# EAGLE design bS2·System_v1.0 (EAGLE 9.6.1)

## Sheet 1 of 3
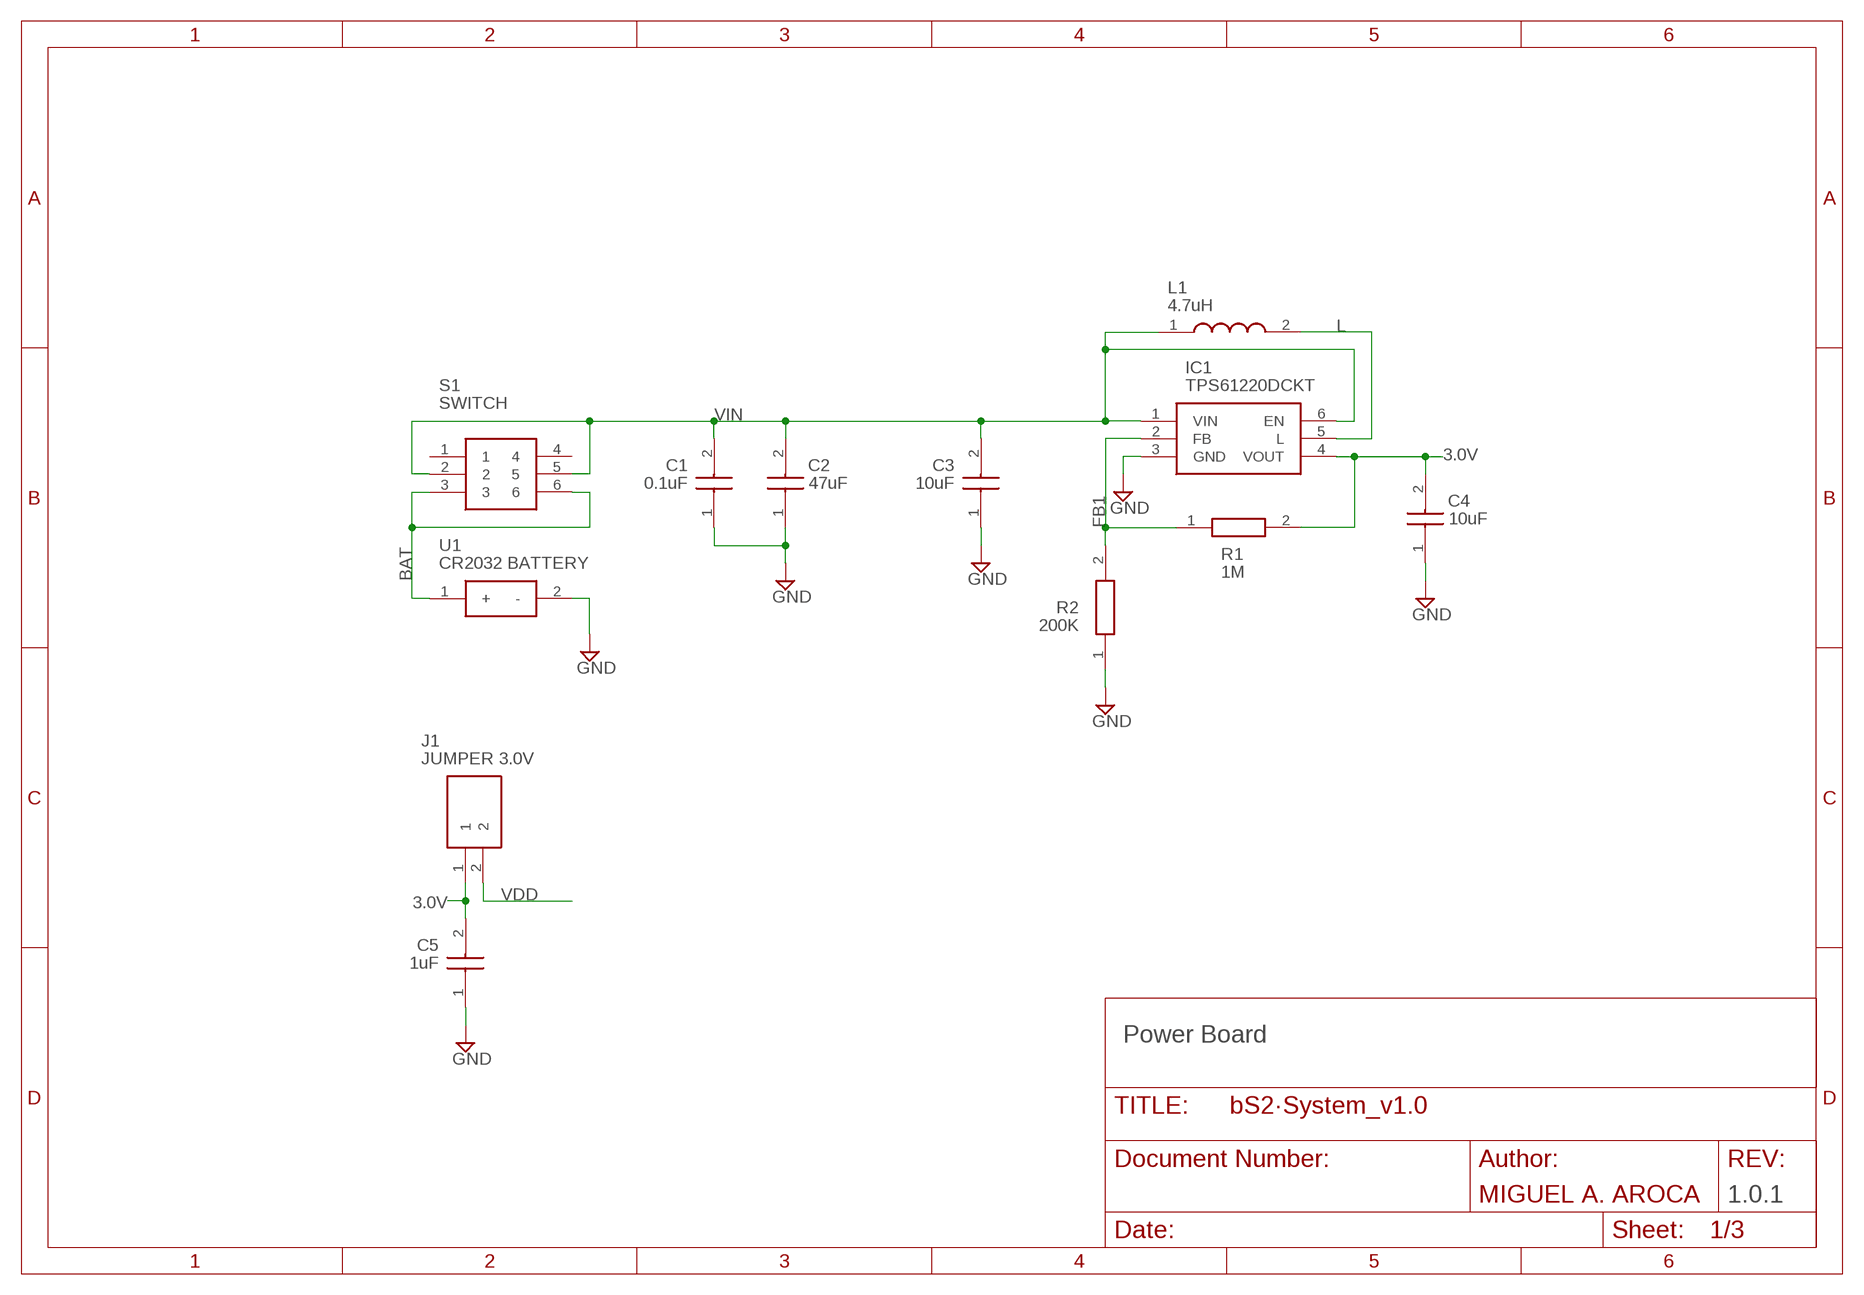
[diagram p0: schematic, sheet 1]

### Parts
C1  0.1uF  C0402C104K4RAC7411  [CAPC1005X55N]
C2  47uF  C1210C476K8RACTU  [CAPC3225X280N]
C3  10uF  GRM188R60J106ME84D  [CAPC1608X90N]
C4  10uF  GRM188R60J106ME84D  [CAPC1608X90N]
C5  1uF  0603ZC105KAT2A  [CAPC1608X90N]
IC1  TPS61220DCKT  [SOT65P210X110-6N]
J1  JUMPER 3.0V  22-28-4027  [HDRV2W66P0X254_1X2_508X249X106]
L1  4.7uH  EPL3015-472MLB  [INDC3030X155N]
R1  1M  CR0402-FX-1004GLF  [RESC1005X40N]
R2  200K  CR0402-JW-204GLF  [RESC1005X40N]
S1  SWITCH  JS202011SCQN  [JS202011SCQN]
U1  CR2032 BATTERY  SMTU2032-LF  [SMTU2032LF]

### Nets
3.0V: C4.2 C5.2 IC1.4(VOUT) J1.1 R1.2
BAT: S1.3 S1.6 U1.1(+)
FB1: IC1.2(FB) R1.1 R2.2
GND: C1.1 C2.1 C3.1 C4.1 C5.1 IC1.3(GND) R2.1 U1.2(-) ; also sheet 2,3
L: IC1.5(L) L1.2
VDD: J1.2 ; also sheet 2,3
VIN: C1.2 C2.2 C3.2 IC1.1(VIN) IC1.6(EN) L1.1 S1.2 S1.5
Unconnected: S1.1 S1.4

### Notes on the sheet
- Power Board
- 1.0.1

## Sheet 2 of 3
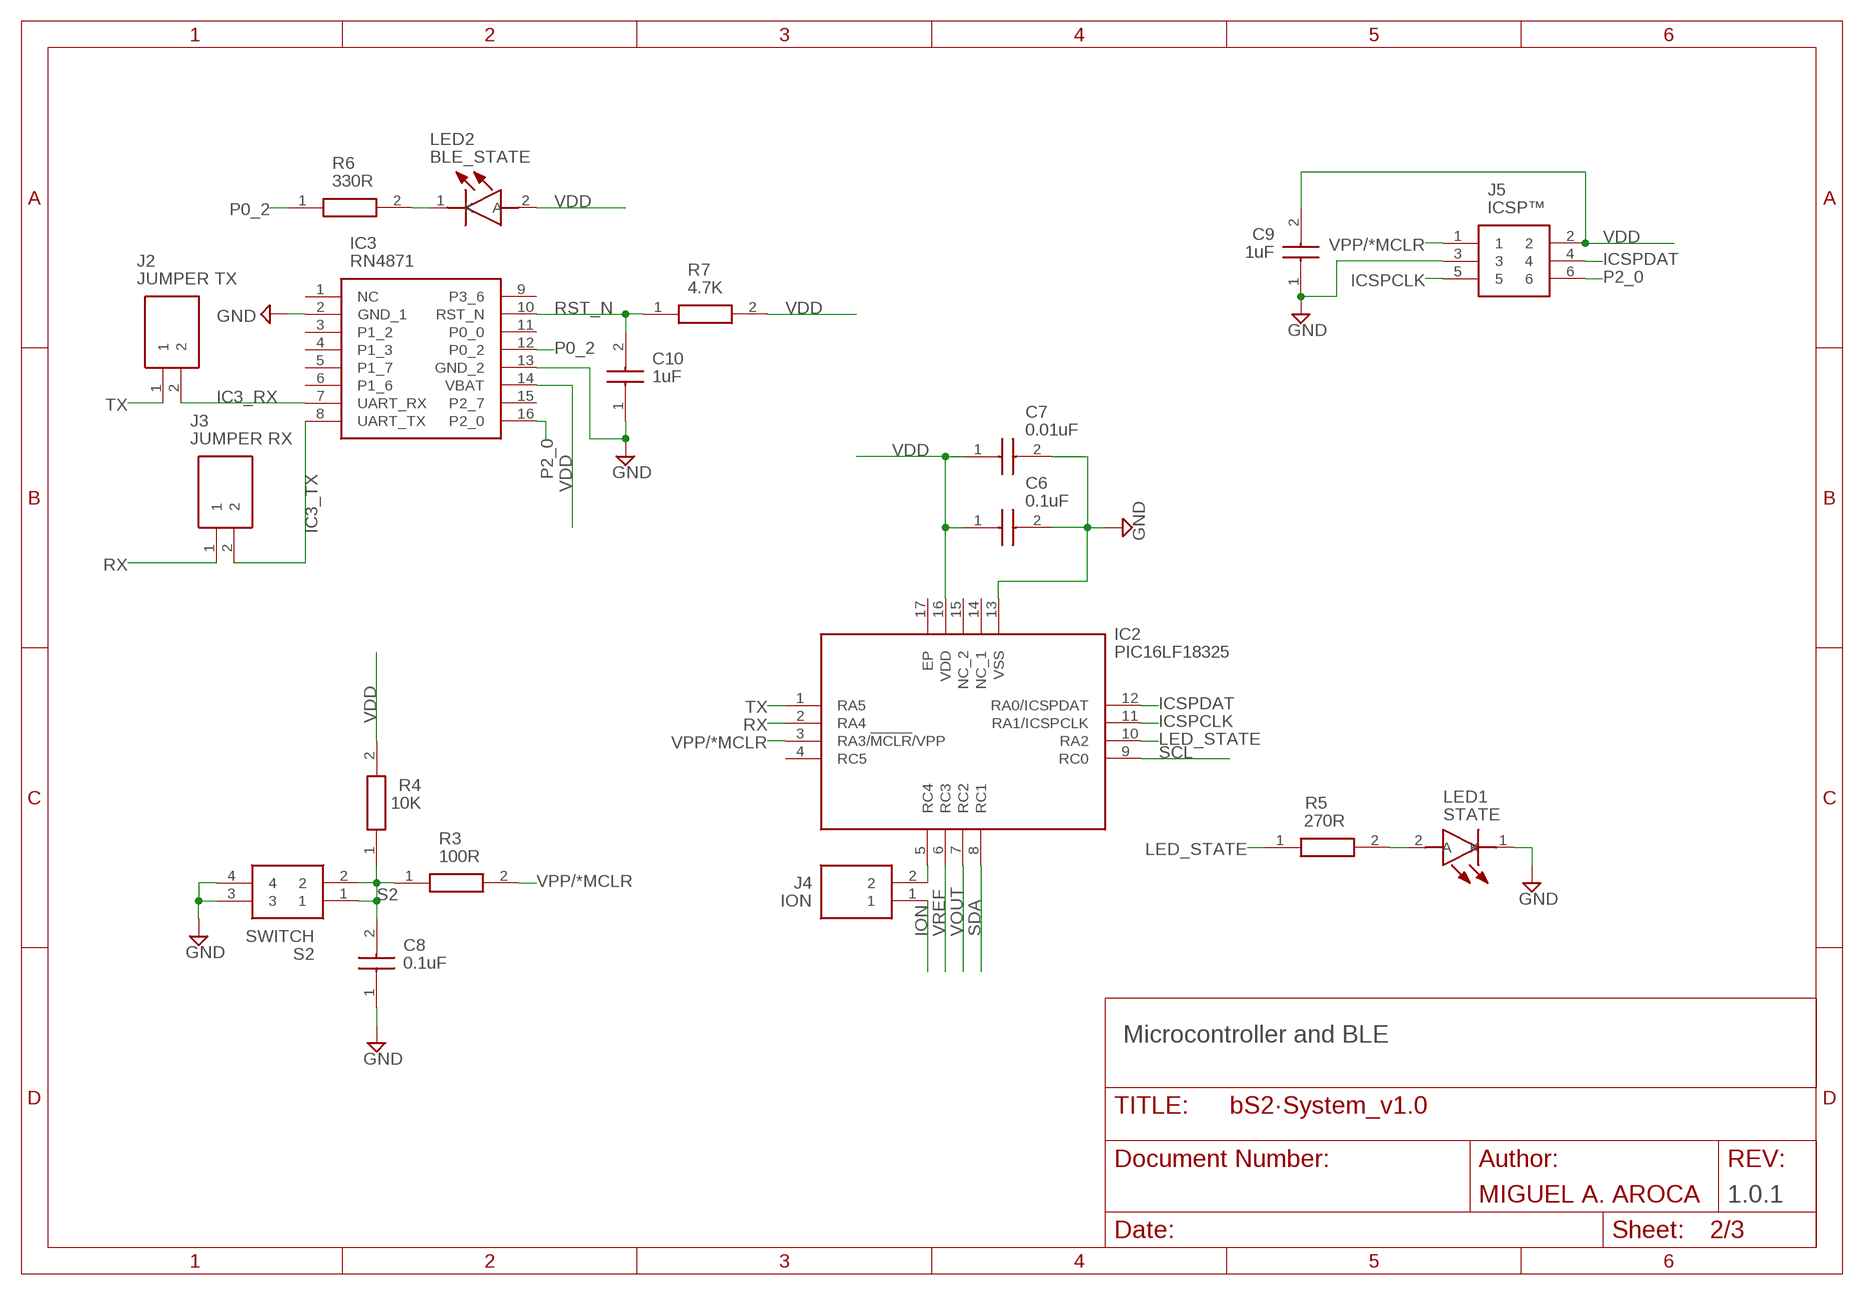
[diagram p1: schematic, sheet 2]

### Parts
C6  0.1uF  C0402C104K4RAC7411  [CAPC1005X55N]
C7  0.01uF  0402ZC103JAT2A  [CAPC1005X56N]
C8  0.1uF  C0402C104K4RAC7411  [CAPC1005X55N]
C9  1uF  0603ZC105KAT2A  [CAPC1608X90N]
C10  1uF  0603ZC105KAT2A  [CAPC1608X90N]
IC2  PIC16LF18325  PIC16LF18325-I_JQ  [QFN65P400X400X55-17N]
IC3  RN4871  RN4871-I_RM130  [RN4871]
J2  JUMPER TX  22-28-4027  [HDRV2W66P0X254_1X2_508X249X106]
J3  JUMPER RX  22-28-4027  [HDRV2W66P0X254_1X2_508X249X106]
J4  ION  22-28-4027  [HDRV2W66P0X254_1X2_508X249X106]
J5  ICSP™  87898-0666  [878980666]
LED1  STATE  SMLP12BC7TT86  [LEDC1006X25N]
LED2  BLE_STATE  SMLP12BC7TT86  [LEDC1006X25N]
R3  100R  CR0402-JW-101GLF  [RESC1005X40N]
R4  10K  CRCW040210K0FKED  [RESC1005X40N]
R5  270R  CR0402-JW-271GLF  [RESC1005X40N]
R6  330R  CR0402-JW-331GLF  [RESC1005X40N]
R7  4.7K  CR0402-JW-472GLF  [RESC1005X40N]
S2  SWITCH  SKRPANE010  [SKRPADE010]

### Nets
GND: C6.2 C7.2 C8.1 C9.1 C10.1 IC2.13(VSS) IC3.2(GND_1) IC3.13(GND_2) J5.3 LED1.1(K) S2.3 S2.4 ; also sheet 1,3
IC3_RX: IC3.7(UART_RX) J2.2
IC3_TX: IC3.8(UART_TX) J3.2
ICSPCLK: IC2.11(RA1/ICSPCLK) J5.5
ICSPDAT: IC2.12(RA0/ICSPDAT) J5.4
ION: J4.1 ; also sheet 3
LED1: LED1.2(A) R5.2
LED2_K: LED2.1(K) R6.2
LED_STATE: IC2.10(RA2) R5.1
P0_2: IC3.12(P0_2) R6.1
P2_0: IC3.16(P2_0) J5.6
RC4: IC2.5(RC4) J4.2
RST_N: C10.2 IC3.10(RST_N) R7.1
RX: IC2.2(RA4) J3.1
S2: C8.2 R3.1 R4.1 S2.1 S2.2
SCL: IC2.9(RC0) ; also sheet 3
SDA: IC2.8(RC1) ; also sheet 3
TX: IC2.1(RA5) J2.1
VDD: C6.1 C7.1 C9.2 IC2.16(VDD) IC3.14(VBAT) J5.2 LED2.2(A) R4.2 R7.2 ; also sheet 1,3
VOUT: IC2.7(RC2) ; also sheet 3
VPP/*MCLR: IC2.3(RA3/!MCLR!/VPP) J5.1 R3.2
VREF: IC2.6(RC3) ; also sheet 3
Unconnected: IC2.4(RC5) IC2.14(NC_1) IC2.15(NC_2) IC2.17(EP) IC3.1(NC) IC3.3(P1_2) IC3.4(P1_3) IC3.5(P1_7) IC3.6(P1_6) IC3.9(P3_6) IC3.11(P0_0) IC3.15(P2_7)

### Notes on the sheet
- Microcontroller and BLE
- 1.0.1

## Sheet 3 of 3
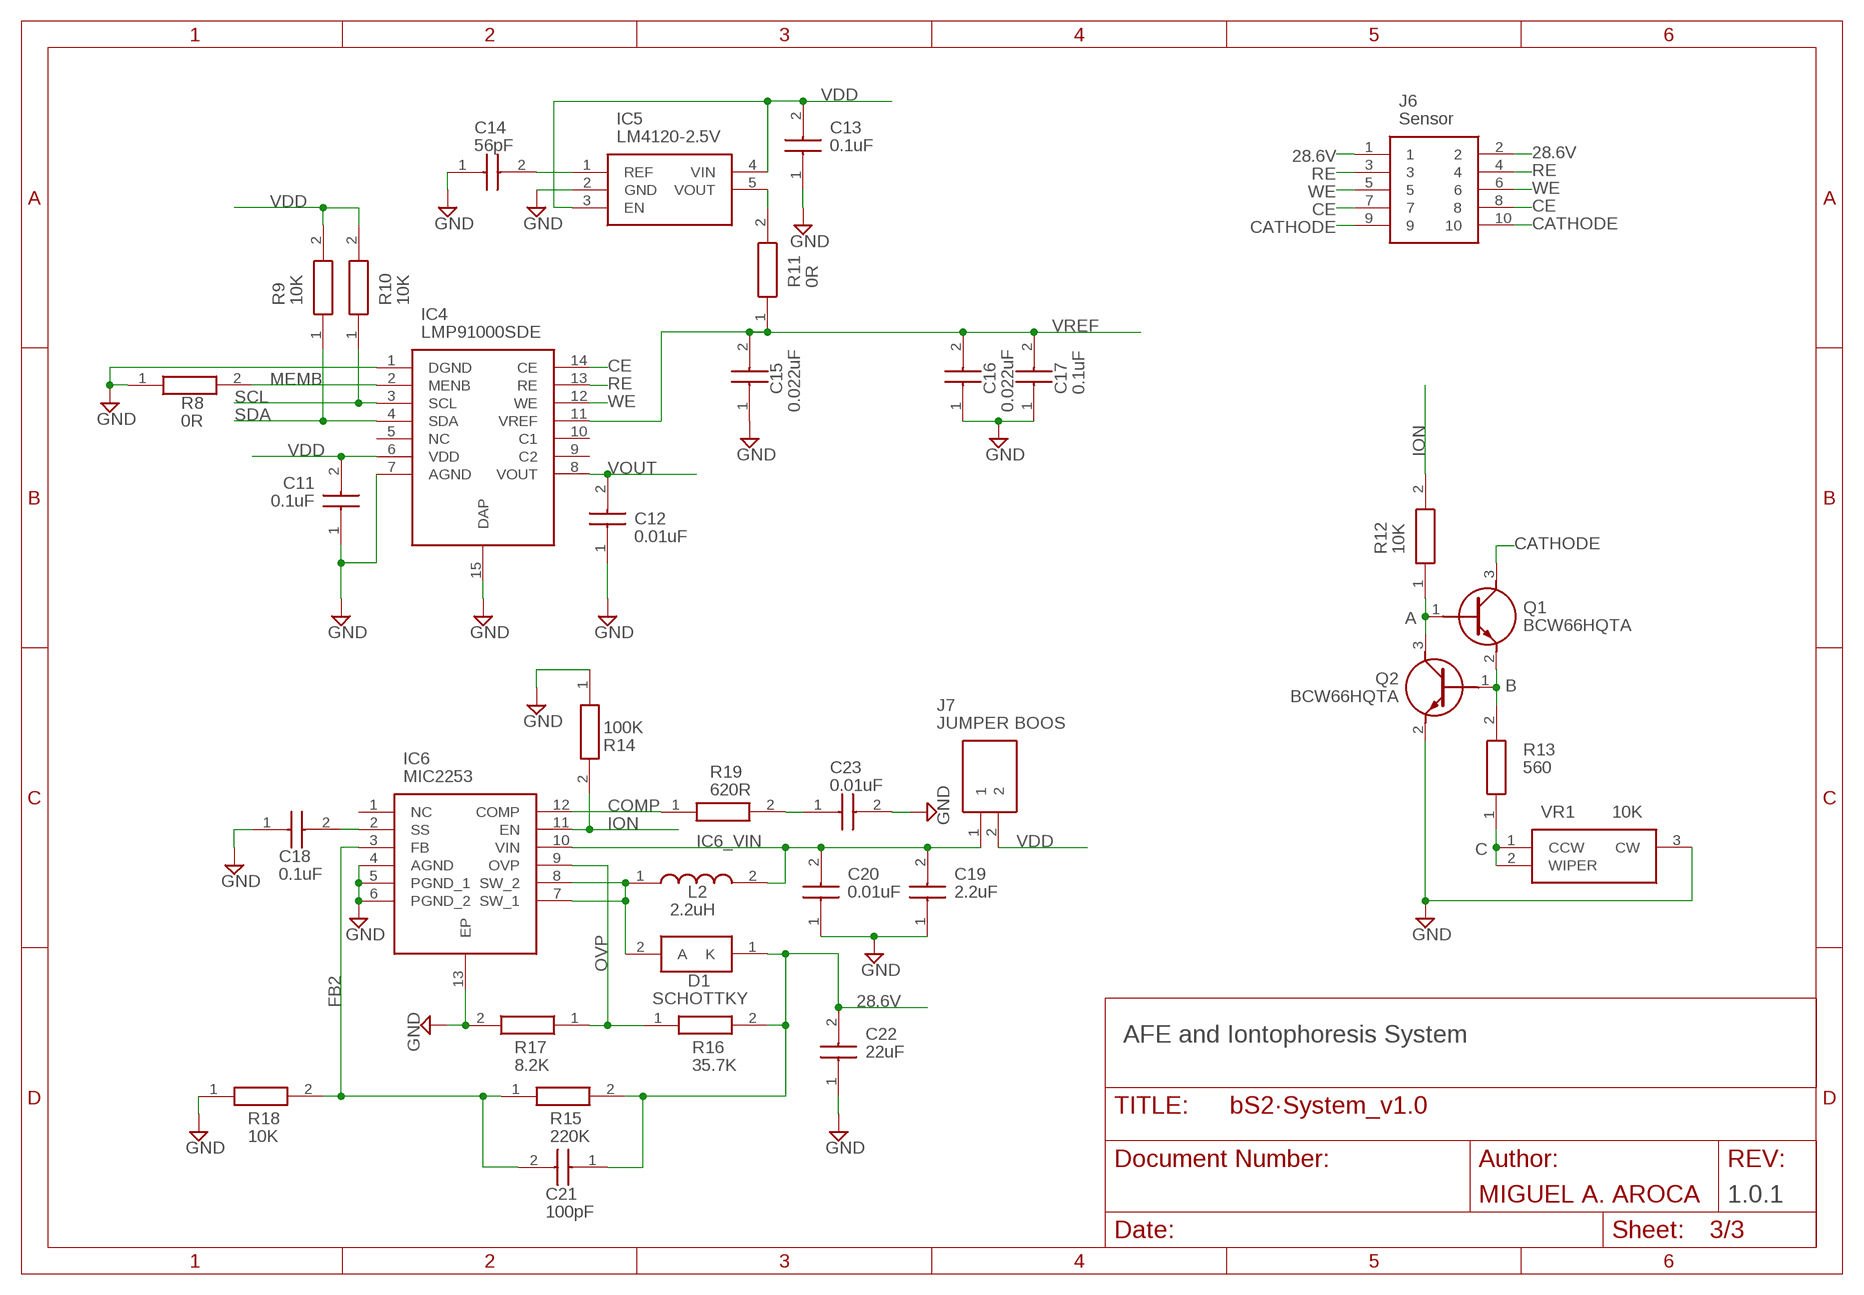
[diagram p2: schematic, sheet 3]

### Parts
C11  0.1uF  C0402C104K4RAC7411  [CAPC1005X55N]
C12  0.01uF  0402ZC103JAT2A  [CAPC1005X56N]
C13  0.1uF  C0402C104K4RAC7411  [CAPC1005X55N]
C14  56pF  VJ0402D560JXAAJ  [CAPC1005X61N]
C15  0.022uF  C0402C223K4RACTU  [CAPC1005X55N]
C16  0.022uF  C0402C223K4RACTU  [CAPC1005X55N]
C17  0.1uF  C0402C104K4RAC7411  [CAPC1005X55N]
C18  0.1uF  CGA2B3X7R1H104K050BE  [CAPC1005X55N]
C19  2.2uF  GRM188R61H225KE11D  [CAPC1608X90N]
C20  0.01uF  C1005X7R1H103K050BE  [CAPC1005X55N]
C21  100pF  C0402C101F5GAC  [CAPC1005X55N]
C22  22uF  C3216X5R1V226M160AC  [CAPC3216X180N]
C23  0.01uF  C1005X7R1H103K050BE  [CAPC1005X55N]
D1  SCHOTTKY  SSA24-E3_61T  [DIONM5127X229N]
IC4  LMP91000SDE  LMP91000SDE_NOPB  [SON50P400X400X80-15N]
IC5  LM4120-2.5V  LM4120AIM5-2.5_NOPB  [SOT95P280X145-5N]
IC6  MIC2253  MIC2253-06YML-TR  [SON50P300X300X90-13N]
J6  Sensor  39-53-2104  [39532104]
J7  JUMPER BOOS  22-28-4027  [HDRV2W66P0X254_1X2_508X249X106]
L2  2.2uH  XAL4020-222MEC  [XAL40XX]
Q1  BCW66HQTA  [FMMT619TA]
Q2  BCW66HQTA  [FMMT619TA]
R8  0R  ERJ-2GE0R00X  [RESC1005X40N]
R9  10K  CRCW040210K0FKED  [RESC1005X40N]
R10  10K  CRCW040210K0FKED  [RESC1005X40N]
R11  0R  ERJ-2GE0R00X  [RESC1005X40N]
R12  10K  CRCW040210K0FKED  [RESC1005X40N]
R13  560  CR0402-JW-561GLF  [RESC1005X40N]
R14  100K  ERJ-3EKF1003V  [RESC1608X55N]
R15  220K  ERJ-3EKF2203V  [RESC1608X55N]
R16  35.7K  ERJ-3EKF3572V  [RESC1608X55N]
R17  8.2K  ERJ-3EKF8201V  [RESC1608X55N]
R18  10K  ERJ-3EKF1002V  [RESC1608X55N]
R19  620R  ERJ-3EKF6200V  [RESC1608X55N]
VR1  10K  3224W-1-103E  [3224W1205E]

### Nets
28.6V: C21.1 C22.2 D1.1(K) J6.1 J6.2 R15.2 R16.2
A: Q1.1(B) Q2.3(C) R12.1
B: Q1.2(E) Q2.1(B) R13.2
C: R13.1 VR1.1(CCW) VR1.2(WIPER)
CATHODE: J6.9 J6.10 Q1.3(C)
CE: IC4.14(CE) J6.7 J6.8
COMP: IC6.12(COMP) R19.1
COMP*: C23.1 R19.2
FB2: C21.2 IC6.3(FB) R15.1 R18.2
GND: C11.1 C12.1 C13.1 C14.1 C15.1 C16.1 C17.1 C18.1 C19.1 C20.1 C22.1 C23.2 IC4.1(DGND) IC4.7(AGND) IC4.15(DAP) IC5.2(GND) IC6.4(AGND) IC6.5(PGND_1) IC6.6(PGND_2) IC6.13(EP) Q2.2(E) R8.1(R1) R14.1 R17.2 R18.1 VR1.3(CW) ; also sheet 1,2
IC5_OUT: IC5.5(VOUT) R11.2(R2)
IC5_REF: C14.2 IC5.1(REF)
IC6_VIN: C19.2 C20.2 IC6.10(VIN) J7.1 L2.2
ION: IC6.11(EN) R12.2 R14.2 ; also sheet 2
MEMB: IC4.2(MENB) R8.2(R2)
OVP: IC6.9(OVP) R16.1 R17.1
RE: IC4.13(RE) J6.3 J6.4
SCL: IC4.3(SCL) R10.1 ; also sheet 2
SDA: IC4.4(SDA) R9.1 ; also sheet 2
SS: C18.2 IC6.2(SS)
SW: D1.2(A) IC6.7(SW_1) IC6.8(SW_2) L2.1
VDD: C11.2 C13.2 IC4.6(VDD) IC5.3(EN) IC5.4(VIN) J7.2 R9.2 R10.2 ; also sheet 1,2
VOUT: C12.2 IC4.8(VOUT) ; also sheet 2
VREF: C15.2 C16.2 C17.2 IC4.11(VREF) R11.1(R1) ; also sheet 2
WE: IC4.12(WE) J6.5 J6.6
Unconnected: IC4.5(NC) IC4.9(C2) IC4.10(C1) IC6.1(NC)

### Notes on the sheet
- AFE and Iontophoresis System
- 1.0.1

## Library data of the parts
C1 C6 C8 C11 C13 C17 = SamacSys_Parts:C0402C104K4RAC7411: Multilayer Ceramic Capacitors MLCC - SMD/SMT 16V 0.1uF X7R 0402 10%; DESCRIPTION: Multilayer Ceramic Capacitors MLCC - SMD/SMT 16V 0.1uF X7R 0402 10%; HEIGHT: 0.55mm; MANUFACTURER_NAME: Kemet; MANUFACTURER_PART_NUMBER: C0402C104K4RAC7411; MOUSER_PART_NUMBER: 80-C0402C104K4R7411; MOUSER_PRICE-STOCK: https://www.mouser.com/Search/Refine.aspx?Keyword=80-C0402C104K4R7411; RS_PART_NUMBER: 1806459; RS_PRICE-STOCK: http://uk.rs-online.com/web/p/products/1806459
C2 = SamacSys_Parts:C1210C476K8RACTU: Multilayer Ceramic Capacitors MLCC - SMD/SMT 10volts 47uF 10% X7R; DESCRIPTION: Multilayer Ceramic Capacitors MLCC - SMD/SMT 10volts 47uF 10% X7R; HEIGHT: 2.8mm; MANUFACTURER_NAME: Kemet; MANUFACTURER_PART_NUMBER: C1210C476K8RACTU; MOUSER_PART_NUMBER: 80-C1210C476K8R; MOUSER_PRICE-STOCK: https://www.mouser.com/Search/Refine.aspx?Keyword=80-C1210C476K8R; RS_PART_NUMBER: 1611519P; RS_PRICE-STOCK: http://uk.rs-online.com/web/p/products/1611519P
C3 C4 = SamacSys_Parts:GRM188R60J106ME84D: Multilayer Ceramic Capacitors MLCC - SMD/SMT 0603 10uF 6.3volts X5R 20%; DESCRIPTION: Multilayer Ceramic Capacitors MLCC - SMD/SMT 0603 10uF 6.3volts X5R 20%; HEIGHT: 0.9mm; MANUFACTURER_NAME: Murata Electronics; MANUFACTURER_PART_NUMBER: GRM188R60J106ME84D; MOUSER_PART_NUMBER: 81-GRM188R60J106ME4D; MOUSER_PRICE-STOCK: https://www.mouser.com/Search/Refine.aspx?Keyword=81-GRM188R60J106ME4D; RS_PART_NUMBER: 8847242P; RS_PRICE-STOCK: http://uk.rs-online.com/web/p/products/8847242P
C5 C9 C10 = SamacSys_Parts:0603ZC105KAT2A: AVX - 0603ZC105KAT2A - CAP, MLCC, X7R, 1UF, 10V, 0603; DESCRIPTION: AVX - 0603ZC105KAT2A - CAP, MLCC, X7R, 1UF, 10V, 0603; HEIGHT: 0.9mm; MANUFACTURER_NAME: AVX; MANUFACTURER_PART_NUMBER: 0603ZC105KAT2A; MOUSER_PART_NUMBER: 581-0603ZC105KAT2A; MOUSER_PRICE-STOCK: https://www.mouser.com/Search/Refine.aspx?Keyword=581-0603ZC105KAT2A; RS_PART_NUMBER: 1358373; RS_PRICE-STOCK: http://uk.rs-online.com/web/p/products/1358373
C7 C12 = SamacSys_Parts:0402ZC103JAT2A: Multilayer Ceramic Capacitors MLCC - SMD/SMT 10V .01uF X7R 0402 5%; DESCRIPTION: Multilayer Ceramic Capacitors MLCC - SMD/SMT 10V .01uF X7R 0402 5%; HEIGHT: 0.56mm; MANUFACTURER_NAME: AVX; MANUFACTURER_PART_NUMBER: 0402ZC103JAT2A; MOUSER_PART_NUMBER: 581-0402ZC103JAT2A; MOUSER_PRICE-STOCK: https://www.mouser.com/Search/Refine.aspx?Keyword=581-0402ZC103JAT2A
C14 = SamacSys_Parts:VJ0402D560JXAAJ: Multilayer Ceramic Capacitors MLCC - SMD/SMT 0402 56pF 50V C0G 5% HI FREQ; DESCRIPTION: Multilayer Ceramic Capacitors MLCC - SMD/SMT 0402 56pF 50V C0G 5% HI FREQ; HEIGHT: 0.61mm; MANUFACTURER_NAME: VISHAY VITRAMON; MANUFACTURER_PART_NUMBER: VJ0402D560JXAAJ
C15 C16 = SamacSys_Parts:C0402C223K4RACTU: Kemet 1005 C0402C 22nF Ceramic Multilayer Capacitor, 16 V dc, +125C, X7R Dielectric, +/-10%; DESCRIPTION: Kemet 1005 C0402C 22nF Ceramic Multilayer Capacitor, 16 V dc, +125C, X7R Dielectric, +/-10%; HEIGHT: 0.55mm; MANUFACTURER_NAME: Kemet; MANUFACTURER_PART_NUMBER: C0402C223K4RACTU; MOUSER_PART_NUMBER: 80-C0402C223K4R; MOUSER_PRICE-STOCK: https://www.mouser.com/Search/Refine.aspx?Keyword=80-C0402C223K4R; RS_PART_NUMBER: 0147724; RS_PRICE-STOCK: http://uk.rs-online.com/web/p/products/0147724
C18 = SamacSys_Parts:CGA2B3X7R1H104K050BE: Multilayer Ceramic Capacitors MLCC - SMD/SMT 0402 0.1uF 50volts X7R 10% Soft Term; DESCRIPTION: Multilayer Ceramic Capacitors MLCC - SMD/SMT 0402 0.1uF 50volts X7R 10% Soft Term; HEIGHT: 0.55mm; MANUFACTURER_NAME: TDK; MANUFACTURER_PART_NUMBER: CGA2B3X7R1H104K050BE; MOUSER_PART_NUMBER: 810-CGA2B3X7R1H104KB; MOUSER_PRICE-STOCK: https://www.mouser.com/Search/Refine.aspx?Keyword=810-CGA2B3X7R1H104KB
C19 = SamacSys_Parts:GRM188R61H225KE11D: Murata 1608 GRM 2200nF Ceramic Multilayer Capacitor, 50 V dc, +85C, X5R Dielectric, +/-10%; DESCRIPTION: Murata 1608 GRM 2200nF Ceramic Multilayer Capacitor, 50 V dc, +85C, X5R Dielectric, +/-10%; HEIGHT: 0.9mm; MANUFACTURER_NAME: Murata Electronics; MANUFACTURER_PART_NUMBER: GRM188R61H225KE11D; MOUSER_PART_NUMBER: 81-GRM188R61H225KE1D; MOUSER_PRICE-STOCK: https://www.mouser.com/Search/Refine.aspx?Keyword=81-GRM188R61H225KE1D; RS_PART_NUMBER: 8847289P; RS_PRICE-STOCK: http://uk.rs-online.com/web/p/products/8847289P
C20 C23 = SamacSys_Parts:C1005X7R1H103K050BE: Multilayer Ceramic Capacitors MLCC - SMD/SMT 0402 0.01uF 50volts X7R 10% Soft Term; DESCRIPTION: Multilayer Ceramic Capacitors MLCC - SMD/SMT 0402 0.01uF 50volts X7R 10% Soft Term; HEIGHT: 0.55mm; MANUFACTURER_NAME: TDK; MANUFACTURER_PART_NUMBER: C1005X7R1H103K050BE; MOUSER_PART_NUMBER: 810-C1005X7R1H103KBE; MOUSER_PRICE-STOCK: https://www.mouser.com/Search/Refine.aspx?Keyword=810-C1005X7R1H103KBE
C21 = SamacSys_Parts:C0402C101F5GAC: Multilayer Ceramic Capacitors MLCC - SMD/SMT 50volts 100pF 1% C0G; DESCRIPTION: Multilayer Ceramic Capacitors MLCC - SMD/SMT 50volts 100pF 1% C0G; HEIGHT: 0.55mm; MANUFACTURER_NAME: Kemet; MANUFACTURER_PART_NUMBER: C0402C101F5GAC; MOUSER_PART_NUMBER: 80-C0402C101F5GAC; MOUSER_PRICE-STOCK: https://www.mouser.com/Search/Refine.aspx?Keyword=80-C0402C101F5GAC
C22 = SamacSys_Parts:C3216X5R1V226M160AC: Multilayer Ceramic Capacitors MLCC - SMD/SMT 1206 22uF 35volts X5R 20%; DESCRIPTION: Multilayer Ceramic Capacitors MLCC - SMD/SMT 1206 22uF 35volts X5R 20%; HEIGHT: 1.8mm; MANUFACTURER_NAME: TDK; MANUFACTURER_PART_NUMBER: C3216X5R1V226M160AC; MOUSER_PART_NUMBER: 810-C3216X5R1V226M; MOUSER_PRICE-STOCK: https://www.mouser.com/Search/Refine.aspx?Keyword=810-C3216X5R1V226M; RS_PART_NUMBER: 7883063P; RS_PRICE-STOCK: http://uk.rs-online.com/web/p/products/7883063P
D1 = SamacSys_Parts:SSA24-E3_61T: Vishay 40V 2A, Diode, 2-Pin DO-214AC SSA24-E3/61T; ALLIED_NUMBER: R1082641; ALLIED_PRICE-STOCK: https://www.alliedelec.com/vishaydale-ssa24-e3-61t/R1082641/; DESCRIPTION: Vishay 40V 2A, Diode, 2-Pin DO-214AC SSA24-E3/61T; HEIGHT: 2.29mm; MANUFACTURER_NAME: Vishay; MANUFACTURER_PART_NUMBER: SSA24-E3/61T; MOUSER_PART_NUMBER: 625-SSA24-E3; MOUSER_PRICE-STOCK: https://www.mouser.com/Search/Refine.aspx?Keyword=625-SSA24-E3; RS_PART_NUMBER: 7103819P; RS_PRICE-STOCK: http://uk.rs-online.com/web/p/products/7103819P
IC1 = SamacSys_Parts:TPS61220DCKT: TPS61220DCKT, Boost Converter, Step Up 0.5A Adjustable, 1.8 5.5 V, 2000 kHz, 6-Pin SC-70 Source: Datasheet; DESCRIPTION: TPS61220DCKT, Boost Converter, Step Up 0.5A Adjustable, 1.8 5.5 V, 2000 kHz, 6-Pin SC-70; HEIGHT: 1.1mm; MANUFACTURER_NAME: Texas Instruments; MANUFACTURER_PART_NUMBER: TPS61220DCKT; MOUSER_PART_NUMBER: 595-TPS61220DCKT; MOUSER_PRICE-STOCK: https://www.mouser.com/Search/Refine.aspx?Keyword=595-TPS61220DCKT; RS_PART_NUMBER: 7094642P; RS_PRICE-STOCK: http://uk.rs-online.com/web/p/products/7094642P
IC2 = SamacSys_Parts:PIC16LF18325-I_JQ: Microchip Technology PIC16LF18325-I/JQ, 8bit 8 bit CPU Microcontroller, 32MHz, 14 kB Flash, 16-Pin UQFN Source: Datasheet; DESCRIPTION: Microchip Technology PIC16LF18325-I/JQ, 8bit 8 bit CPU Microcontroller, 32MHz, 14 kB Flash, 16-Pin UQFN; HEIGHT: 0.55mm; MANUFACTURER_NAME: Microchip; MANUFACTURER_PART_NUMBER: PIC16LF18325-I/JQ; MOUSER_PART_NUMBER: 579-PIC16LF18325I/JQ; MOUSER_PRICE-STOCK: https://www.mouser.com/Search/Refine.aspx?Keyword=579-PIC16LF18325I%2FJQ; RS_PART_NUMBER: 1772711P; RS_PRICE-STOCK: http://uk.rs-online.com/web/p/products/1772711P
IC3 = SamacSys_Parts:RN4871-I_RM130: Bluetooth BLE Module, Shielded, Antenna, Source: Datasheet; DESCRIPTION: Bluetooth BLE Module, Shielded, Antenna,; HEIGHT: mm; MANUFACTURER_NAME: Microchip; MANUFACTURER_PART_NUMBER: RN4871-I/RM130; MOUSER_PART_NUMBER: 579-RN4871IRM130; MOUSER_PRICE-STOCK: https://www.mouser.com/Search/Refine.aspx?Keyword=579-RN4871IRM130; RS_PART_NUMBER: 1765558P; RS_PRICE-STOCK: http://uk.rs-online.com/web/p/products/1765558P
IC4 = SamacSys_Parts:LMP91000SDE_NOPB: Texas Instruments,LMP91000SDE/NOPB,AFE LMP91000SDE/NOPB, Analogue Front End IC, 1-channel Serial-I2C, 14-Pin WSON Source: Datasheet; DESCRIPTION: Texas Instruments,LMP91000SDE/NOPB,AFE LMP91000SDE/NOPB, Analogue Front End IC, 1-channel Serial-I2C, 14-Pin WSON; HEIGHT: 0.8mm; MANUFACTURER_NAME: Texas Instruments; MANUFACTURER_PART_NUMBER: LMP91000SDE/NOPB; MOUSER_PART_NUMBER: 926-LMP91000SDE/NOPB; MOUSER_PRICE-STOCK: https://www.mouser.com/Search/Refine.aspx?Keyword=926-LMP91000SDE%2FNOPB; RS_PART_NUMBER: 7988774P; RS_PRICE-STOCK: http://uk.rs-online.com/web/p/products/7988774P
IC5 = SamacSys_Parts:LM4120AIM5-2.5_NOPB: 0.2% 50ppm/C Drift Precision Series Voltage Reference with Shutdown Enable Source: Datasheet; DESCRIPTION: 0.2% 50ppm/C Drift Precision Series Voltage Reference with Shutdown Enable; HEIGHT: 1.45mm; MANUFACTURER_NAME: Texas Instruments; MANUFACTURER_PART_NUMBER: LM4120AIM5-2.5/NOPB; MOUSER_PART_NUMBER: 926-LM4120AIM525NOPB; MOUSER_PRICE-STOCK: https://www.mouser.com/Search/Refine.aspx?Keyword=926-LM4120AIM525NOPB; RS_PART_NUMBER: 6394496; RS_PRICE-STOCK: https://uk.rs-online.com/web/p/products/6394496
IC6 = SamacSys_Parts:MIC2253-06YML-TR: 3.5A 1MHz Efficiency Boost Regulator Source: Datasheet; DESCRIPTION: 3.5A 1MHz Efficiency Boost Regulator; HEIGHT: 0.9mm; MANUFACTURER_NAME: Microchip; MANUFACTURER_PART_NUMBER: MIC2253-06YML-TR; MOUSER_PART_NUMBER: 998-MIC2253-06YMLTR; RS_PART_NUMBER: 9101638P; RS_PRICE-STOCK: http://uk.rs-online.com/web/p/products/9101638P
J1-J4 J7 = SamacSys_Parts:22-28-4027: Headers & Wire Housings VERT B/A HDR 2P; ALLIED_NUMBER: 71457608; ALLIED_PRICE-STOCK: https://www.alliedelec.com/molexincorporated-22-28-4027/71457608/; DESCRIPTION: Headers & Wire Housings VERT B/A HDR 2P; HEIGHT: 10.67mm; MANUFACTURER_NAME: Molex; MANUFACTURER_PART_NUMBER: 22-28-4027; MOUSER_PART_NUMBER: 538-22-28-4027; MOUSER_PRICE-STOCK: https://www.mouser.com/Search/Refine.aspx?Keyword=538-22-28-4027
J5 = SamacSys_Parts:87898-0666: Headers & Wire Housings 2.54mm SRSW SMT Hdr W/O Cap 2.5SnLF 6Ckt Source: Datasheet; DESCRIPTION: Headers & Wire Housings 2.54mm SRSW SMT Hdr W/O Cap 2.5SnLF 6Ckt; HEIGHT: 13.1mm; MANUFACTURER_NAME: Molex; MANUFACTURER_PART_NUMBER: 87898-0666; MOUSER_PART_NUMBER: 538-87898-0666; MOUSER_PRICE-STOCK: https://www.mouser.com/Search/Refine.aspx?Keyword=538-87898-0666
J6 = SamacSys_Parts:39-53-2104: Molex FFC/FPC THROUGH HOLE Series 1.25mm Pitch 10 Way Right Angle Female FPC Connector, ZIF Top Contact Source: Datasheet; DESCRIPTION: Molex FFC/FPC THROUGH HOLE Series 1.25mm Pitch 10 Way Right Angle Female FPC Connector, ZIF Top Contact; HEIGHT: 5mm; MANUFACTURER_NAME: Molex; MANUFACTURER_PART_NUMBER: 39-53-2104; MOUSER_PART_NUMBER: 538-39-53-2104; MOUSER_PRICE-STOCK: https://www.mouser.com/Search/Refine.aspx?Keyword=538-39-53-2104; RS_PART_NUMBER: 1671838; RS_PRICE-STOCK: https://uk.rs-online.com/web/p/products/1671838
L1 = SamacSys_Parts:EPL3015-472MLB: Fixed Inductors EPL3015 Low Profile 4.7 uH 20 % 1.4 A; DESCRIPTION: Fixed Inductors EPL3015 Low Profile 4.7 uH 20 % 1.4 A; HEIGHT: 1.55mm; MANUFACTURER_NAME: COILCRAFT; MANUFACTURER_PART_NUMBER: EPL3015-472MLB; MOUSER_PART_NUMBER: 994-EPL3015-472MLB; MOUSER_PRICE-STOCK: https://www.mouser.com/Search/Refine.aspx?Keyword=994-EPL3015-472MLB
L2 = SamacSys_Parts:XAL4020-222MEC: COILCRAFT - XAL4020-222MEC - INDUCTOR, 2.2UH, 5.5A, 20%, PWR, 52MHZ; DESCRIPTION: COILCRAFT - XAL4020-222MEC - INDUCTOR, 2.2UH, 5.5A, 20%, PWR, 52MHZ; HEIGHT: mm; MANUFACTURER_NAME: COILCRAFT; MANUFACTURER_PART_NUMBER: XAL4020-222MEC; MOUSER_PART_NUMBER: 994-XAL4020-222MEC; MOUSER_PRICE-STOCK: https://www.mouser.com/Search/Refine.aspx?Keyword=994-XAL4020-222MEC
LED1 LED2 = SamacSys_Parts:SMLP12BC7TT86: ROHM SMLP12BC7TT86, SML-P12 PICOLED Series Blue LED, 1006 (0402), Rectangle Lens SMD package; DESCRIPTION: ROHM SMLP12BC7TT86, SML-P12 PICOLED Series Blue LED, 1006 (0402), Rectangle Lens SMD package; HEIGHT: 0.25mm; MANUFACTURER_NAME: ROHM Semiconductor; MANUFACTURER_PART_NUMBER: SMLP12BC7TT86; MOUSER_PART_NUMBER: 755-SMLP12BC7TT86; MOUSER_PRICE-STOCK: https://www.mouser.com/Search/Refine.aspx?Keyword=755-SMLP12BC7TT86; RS_PART_NUMBER: 7003589P; RS_PRICE-STOCK: http://uk.rs-online.com/web/p/products/7003589P
Q1 Q2 = SamacSys_Parts:BCW66HQTA: Bipolar Transistors - BJT General Purpose Transistor Source: Datasheet; DESCRIPTION: Bipolar Transistors - BJT General Purpose Transistor; HEIGHT: mm; MANUFACTURER_NAME: Diodes Inc.; MANUFACTURER_PART_NUMBER: BCW66HQTA; MOUSER_PART_NUMBER: 621-BCW66HQTA; MOUSER_PRICE-STOCK: https://www.mouser.com/Search/Refine.aspx?Keyword=621-BCW66HQTA
R1 = SamacSys_Parts:CR0402-FX-1004GLF: Thick Film Resistors - SMD 1.0M OHM 1%; DESCRIPTION: Thick Film Resistors - SMD 1.0M OHM 1%; HEIGHT: 0.4mm; MANUFACTURER_NAME: Bourns; MANUFACTURER_PART_NUMBER: CR0402-FX-1004GLF; MOUSER_PART_NUMBER: 652-CR0402FX-1004GLF; MOUSER_PRICE-STOCK: https://www.mouser.com/Search/Refine.aspx?Keyword=652-CR0402FX-1004GLF
R2 = SamacSys_Parts:CR0402-JW-204GLF: Thick Film Resistors - SMD 200KOHM 1/16WATT 5%; DESCRIPTION: Thick Film Resistors - SMD 200KOHM 1/16WATT 5%; HEIGHT: 0.4mm; MANUFACTURER_NAME: Bourns; MANUFACTURER_PART_NUMBER: CR0402-JW-204GLF; MOUSER_PART_NUMBER: 652-CR0402-JW-204GLF; MOUSER_PRICE-STOCK: https://www.mouser.com/Search/Refine.aspx?Keyword=652-CR0402-JW-204GLF
R3 = SamacSys_Parts:CR0402-JW-101GLF: Bourns Chip Resistors CR0402 series VALUE1; DESCRIPTION: Bourns Chip Resistors CR0402 series VALUE1; HEIGHT: 0.4mm; MANUFACTURER_NAME: Bourns; MANUFACTURER_PART_NUMBER: CR0402-JW-101GLF; MOUSER_PART_NUMBER: 652-CR0402JW-101GLF; MOUSER_PRICE-STOCK: https://www.mouser.com/Search/Refine.aspx?Keyword=652-CR0402JW-101GLF
R4 R9 R10 R12 = SamacSys_Parts:CRCW040210K0FKED: CRCW0402 Resistor T/R 0.063W,1%,10K Vishay CRCW Series Thick Film Surface Mount Resistor 0402 Case 10k +/-1% 0.063W +/-100ppm/C; ALLIED_NUMBER: 70202520; ALLIED_PRICE-STOCK: http://www.alliedelec.com/vishay-dale-crcw040210k0fked/70202520/; DESCRIPTION: CRCW0402 Resistor T/R 0.063W,1%,10K Vishay CRCW Series Thick Film Surface Mount Resistor 0402 Case 10k +/-1% 0.063W +/-100ppm/C; HEIGHT: 0.4mm; MANUFACTURER_NAME: Vishay; MANUFACTURER_PART_NUMBER: CRCW040210K0FKED; MOUSER_PART_NUMBER: 71-CRCW0402-10K-E3; MOUSER_PRICE-STOCK: https://www.mouser.com/Search/Refine.aspx?Keyword=71-CRCW0402-10K-E3; RS_PART_NUMBER: 6784697P; RS_PRICE-STOCK: http://uk.rs-online.com/web/p/products/6784697P
R5 = SamacSys_Parts:CR0402-JW-271GLF: Thick Film Resistors - SMD 270OHM 1/16WATT 5%; DESCRIPTION: Thick Film Resistors - SMD 270OHM 1/16WATT 5%; HEIGHT: 0.4mm; MANUFACTURER_NAME: Bourns; MANUFACTURER_PART_NUMBER: CR0402-JW-271GLF; MOUSER_PART_NUMBER: 652-CR0402-JW-271GLF; MOUSER_PRICE-STOCK: https://www.mouser.com/Search/Refine.aspx?Keyword=652-CR0402-JW-271GLF
R6 = SamacSys_Parts:CR0402-JW-331GLF: Thick Film Resistors - SMD 330 OHM 5%; DESCRIPTION: Thick Film Resistors - SMD 330 OHM 5%; HEIGHT: 0.4mm; MANUFACTURER_NAME: Bourns; MANUFACTURER_PART_NUMBER: CR0402-JW-331GLF; MOUSER_PART_NUMBER: 652-CR0402JW-331GLF; MOUSER_PRICE-STOCK: https://www.mouser.com/Search/Refine.aspx?Keyword=652-CR0402JW-331GLF
R7 = SamacSys_Parts:CR0402-JW-472GLF: BOURNS - CR0402-JW-472GLF - RES, THICK FILM, 4K7, 5%, 0.0625W, 0402; DESCRIPTION: BOURNS - CR0402-JW-472GLF - RES, THICK FILM, 4K7, 5%, 0.0625W, 0402; HEIGHT: 0.4mm; MANUFACTURER_NAME: Bourns; MANUFACTURER_PART_NUMBER: CR0402-JW-472GLF; MOUSER_PART_NUMBER: 652-CR0402-JW-472GLF; MOUSER_PRICE-STOCK: https://www.mouser.com/Search/Refine.aspx?Keyword=652-CR0402-JW-472GLF
R8 R11 = SamacSys_Parts:ERJ-2GE0R00X: RESISTOR, 0402 0 Ohm - 0.1 W; ALLIED_NUMBER: 70264913; ALLIED_PRICE-STOCK: https://www.alliedelec.com/panasonic-erj-2ge0r00x/70264913/; DESCRIPTION: RESISTOR, 0402 0 Ohm - 0.1 W; HEIGHT: mm; MANUFACTURER_NAME: Panasonic; MANUFACTURER_PART_NUMBER: ERJ-2GE0R00X; MOUSER_PART_NUMBER: 667-ERJ-2GE0R00X; MOUSER_PRICE-STOCK: https://www.mouser.com/Search/Refine.aspx?Keyword=667-ERJ-2GE0R00X
R13 = SamacSys_Parts:CR0402-JW-561GLF: Bourns Chip Resistors CR0402 series 561; DESCRIPTION: Bourns Chip Resistors CR0402 series 561; HEIGHT: 0.4mm; MANUFACTURER_NAME: Bourns; MANUFACTURER_PART_NUMBER: CR0402-JW-561GLF; MOUSER_PART_NUMBER: 652-CR0402JW-561GLF; MOUSER_PRICE-STOCK: https://www.mouser.com/Search/Refine.aspx?Keyword=652-CR0402JW-561GLF
R14 = SamacSys_Parts:ERJ-3EKF1003V: Thick Film Resistors - SMD 0603 100Kohms 1% Tol; ALLIED_NUMBER: 70264549; ALLIED_PRICE-STOCK: https://www.alliedelec.com/panasonic-erj-3ekf1003v/70264549/; DESCRIPTION: Thick Film Resistors - SMD 0603 100Kohms 1% Tol; HEIGHT: 0.55mm; MANUFACTURER_NAME: Panasonic; MANUFACTURER_PART_NUMBER: ERJ-3EKF1003V; MOUSER_PART_NUMBER: 667-ERJ-3EKF1003V; MOUSER_PRICE-STOCK: https://www.mouser.com/Search/Refine.aspx?Keyword=667-ERJ-3EKF1003V
R15 = SamacSys_Parts:ERJ-3EKF2203V: RESISTOR, 0603 220 kOhm +/-1 % 0.1 W; ALLIED_NUMBER: 70265715; ALLIED_PRICE-STOCK: https://www.alliedelec.com/panasonic-erj-3ekf2203v/70265715/; DESCRIPTION: RESISTOR, 0603 220 kOhm +/-1 % 0.1 W; HEIGHT: 0.55mm; MANUFACTURER_NAME: Panasonic; MANUFACTURER_PART_NUMBER: ERJ-3EKF2203V; MOUSER_PART_NUMBER: 667-ERJ-3EKF2203V; MOUSER_PRICE-STOCK: https://www.mouser.com/Search/Refine.aspx?Keyword=667-ERJ-3EKF2203V
R16 = SamacSys_Parts:ERJ-3EKF3572V: Thick Film Resistors - SMD 0603 35.7Kohms 1% AEC-Q200; ALLIED_NUMBER: 70265791; ALLIED_PRICE-STOCK: https://www.alliedelec.com/panasonic-erj-3ekf3572v/70265791/; DESCRIPTION: Thick Film Resistors - SMD 0603 35.7Kohms 1% AEC-Q200; HEIGHT: 0.55mm; MANUFACTURER_NAME: Panasonic; MANUFACTURER_PART_NUMBER: ERJ-3EKF3572V; MOUSER_PART_NUMBER: 667-ERJ-3EKF3572V; MOUSER_PRICE-STOCK: https://www.mouser.com/Search/Refine.aspx?Keyword=667-ERJ-3EKF3572V
R17 = SamacSys_Parts:ERJ-3EKF8201V: RESISTOR, 0603 8.2 kOhm +/-1 % 0.1 W; ALLIED_NUMBER: 70265907; ALLIED_PRICE-STOCK: https://www.alliedelec.com/panasonic-erj-3ekf8201v/70265907/; DESCRIPTION: RESISTOR, 0603 8.2 kOhm +/-1 % 0.1 W; HEIGHT: 0.55mm; MANUFACTURER_NAME: Panasonic; MANUFACTURER_PART_NUMBER: ERJ-3EKF8201V; MOUSER_PART_NUMBER: 667-ERJ-3EKF8201V; MOUSER_PRICE-STOCK: https://www.mouser.com/Search/Refine.aspx?Keyword=667-ERJ-3EKF8201V
R18 = SamacSys_Parts:ERJ-3EKF1002V: Thick Film Resistors - SMD 0603 10Kohms 1% AEC-Q200; ALLIED_NUMBER: 70265620; ALLIED_PRICE-STOCK: https://www.alliedelec.com/panasonic-erj-3ekf1002v/70265620/; DESCRIPTION: Thick Film Resistors - SMD 0603 10Kohms 1% AEC-Q200; HEIGHT: 0.55mm; MANUFACTURER_NAME: Panasonic; MANUFACTURER_PART_NUMBER: ERJ-3EKF1002V; MOUSER_PART_NUMBER: 667-ERJ-3EKF1002V; MOUSER_PRICE-STOCK: https://www.mouser.com/Search/Refine.aspx?Keyword=667-ERJ-3EKF1002V
R19 = SamacSys_Parts:ERJ-3EKF6200V: Thick Film Resistors - SMD 0603 620ohms 1% AEC-Q200; ALLIED_NUMBER: 70269499; ALLIED_PRICE-STOCK: https://www.alliedelec.com/panasonic-erj-3ekf6200v/70269499/; DESCRIPTION: Thick Film Resistors - SMD 0603 620ohms 1% AEC-Q200; HEIGHT: 0.55mm; MANUFACTURER_NAME: Panasonic; MANUFACTURER_PART_NUMBER: ERJ-3EKF6200V; MOUSER_PART_NUMBER: 667-ERJ-3EKF6200V; MOUSER_PRICE-STOCK: https://www.mouser.com/Search/Refine.aspx?Keyword=667-ERJ-3EKF6200V
S1 = SamacSys_Parts:JS202011SCQN: Sub miniature slide switches Source: Datasheet; DESCRIPTION: Sub miniature slide switches; HEIGHT: mm; MANUFACTURER_NAME: C & K COMPONENTS; MANUFACTURER_PART_NUMBER: JS202011SCQN; MOUSER_PART_NUMBER: 611-JS202011SCQN; MOUSER_PRICE-STOCK: https://www.mouser.com/Search/Refine.aspx?Keyword=611-JS202011SCQN; RS_PART_NUMBER: 1546137; RS_PRICE-STOCK: http://uk.rs-online.com/web/p/products/1546137
S2 = SamacSys_Parts:SKRPANE010: Tactile Switches 500mOhm 1.57N 16VDC 4.2X3.2X2.5MM 50mA Source: Datasheet; DESCRIPTION: Tactile Switches 500mOhm 1.57N 16VDC 4.2X3.2X2.5MM 50mA; HEIGHT: 2mm; MANUFACTURER_NAME: ALPS; MANUFACTURER_PART_NUMBER: SKRPANE010; MOUSER_PART_NUMBER: 688-SKRPANE010; MOUSER_PRICE-STOCK: https://www.mouser.com/Search/Refine.aspx?Keyword=688-SKRPANE010
U1 = SamacSys_Parts:SMTU2032-LF: Coin Cell Battery Holders SFC MNT FOR CR2032; DESCRIPTION: Coin Cell Battery Holders SFC MNT FOR CR2032; HEIGHT: 5mm; MANUFACTURER_NAME: RENATA; MANUFACTURER_PART_NUMBER: SMTU2032-LF; MOUSER_PART_NUMBER: 614-SMTU2032-LF; MOUSER_PRICE-STOCK: https://www.mouser.com/Search/Refine.aspx?Keyword=614-SMTU2032-LF
VR1 = SamacSys_Parts:3224W-1-103E: Bourns 3224W Series 12-Turn SMD Cermet Trimmer Resistor with J-Hook Terminations, 10000 +/-10% 0.25W +/-100ppm/C Source: Datasheet; ALLIED_NUMBER: 70153354; ALLIED_PRICE-STOCK: https://www.alliedelec.com/bourns-3224w-1-103e/70153354/; DESCRIPTION: Bourns 3224W Series 12-Turn SMD Cermet Trimmer Resistor with J-Hook Terminations, 10000 +/-10% 0.25W +/-100ppm/C; HEIGHT: 5mm; MANUFACTURER_NAME: Bourns; MANUFACTURER_PART_NUMBER: 3224W-1-103E; MOUSER_PART_NUMBER: 652-3224W-1-103E; MOUSER_PRICE-STOCK: https://www.mouser.com/Search/Refine.aspx?Keyword=652-3224W-1-103E; RS_PART_NUMBER: 0177481P; RS_PRICE-STOCK: http://uk.rs-online.com/web/p/products/0177481P

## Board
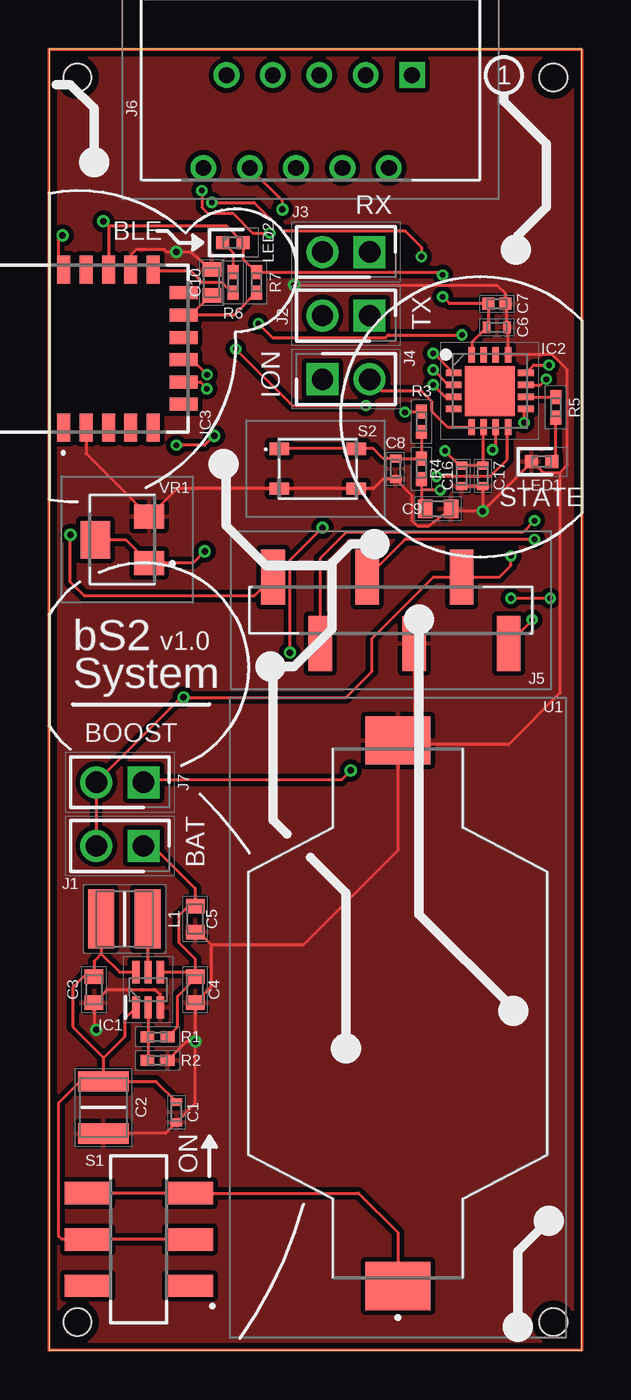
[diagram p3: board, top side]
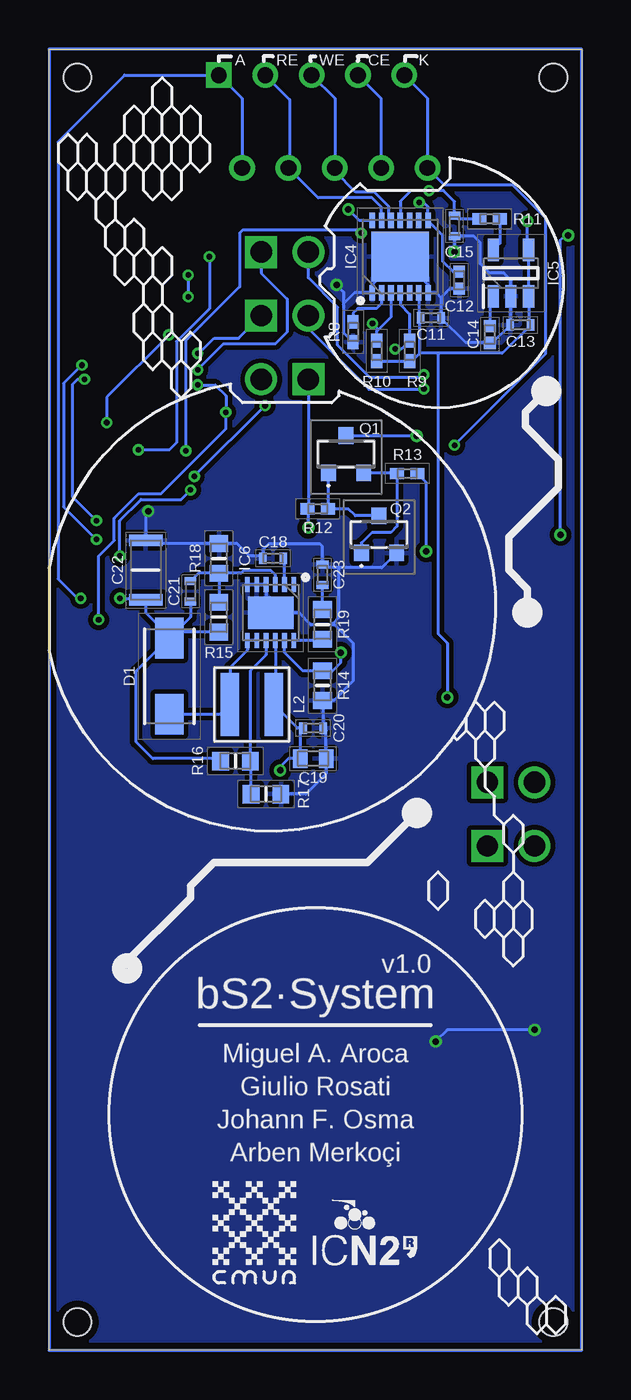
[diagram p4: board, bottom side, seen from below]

Size 28.7 x 70.1 mm. Coordinates in mm from the lower left corner, seen from the top.
Outline: 0,0 28.7,0 28.7,70.1 0,70.1 0,0
Copper layers (1*16): Top 0.035mm / dielectric 1.5mm / Bottom 0.035mm
Design rules "PCBWay - 2 CAPAS *": minimum track width 6mil, minimum drill 0.3mm, track to track 6mil, track to pad 6mil, pad to pad 6mil, via to via 6mil, smd to smd 6mil, copper to edge 0.4mm, drill to drill 0.2mm, minimum pad ring 6mil, minimum via ring 6mil, stop-mask expansion 2mil, vias tented up to drill 0mil, thermal gap 10mil
Holes 1.5 mm at 1.52,68.58 27.18,68.58 27.18,1.52 1.52,1.52

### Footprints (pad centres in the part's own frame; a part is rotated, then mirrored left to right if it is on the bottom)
CAPC1005X55N = smd 0.42 x 0.62: 1 -0.55,0; 2 0.55,0
CAPC3225X280N = smd 1.1 x 2.74: 1 -1.41,0; 2 1.41,0
CAPC1608X90N = smd 0.78 x 0.99: 1 -0.7,0; 2 0.7,0
CAPC1005X56N = smd 0.65 x 0.64: 1 -0.45,0; 2 0.45,0
CAPC1005X61N = smd 0.66 x 0.65: 1 -0.45,0; 2 0.45,0
CAPC3216X180N = smd 0.62 x 1.82: 1 -1.6,0; 2 1.6,0
DIONM5127X229N = smd 2.2 x 1.55: 1 -2.05,0; 2 2.05,0
SOT65P210X110-6N = smd 1.2 x 0.4: 1 -0.95,0.65; 2 -0.95,0; 3 -0.95,-0.65; 4 0.95,-0.65; 5 0.95,0; 6 0.95,0.65
QFN65P400X400X55-17N = smd 0.85 x 0.35: 1 -1.95,0.975; 2 -1.95,0.325; 3 -1.95,-0.325; 4 -1.95,-0.975; 9 1.95,-0.975; 10 1.95,-0.325; 11 1.95,0.325; 12 1.95,0.975 | smd 0.35 x 0.85: 5 -0.975,-1.95; 6 -0.325,-1.95; 7 0.325,-1.95; 8 0.975,-1.95; 13 0.975,1.95; 14 0.325,1.95; 15 -0.325,1.95; 16 -0.975,1.95 | smd 2.7 x 2.7: 17 0,0
RN4871 = smd 1.5 x 0.7: 1 -4.25,6.7; 2 -4.25,5.5; 3 -4.25,4.3; 4 -4.25,3.1; 5 -4.25,1.9; 12 4.25,1.9; 13 4.25,3.1; 14 4.25,4.3; 15 4.25,5.5; 16 4.25,6.7 | smd 0.7 x 1.5: 6 -3,0.25; 7 -1.8,0.25; 8 -0.6,0.25; 9 0.6,0.25; 10 1.8,0.25; 11 3,0.25
SON50P400X400X80-15N = smd 0.85 x 0.3: 1 -1.95,1.5; 2 -1.95,1; 3 -1.95,0.5; 4 -1.95,0; 5 -1.95,-0.5; 6 -1.95,-1; 7 -1.95,-1.5; 8 1.95,-1.5; 9 1.95,-1; 10 1.95,-0.5; 11 1.95,0; 12 1.95,0.5; 13 1.95,1; 14 1.95,1.5 | smd 2.7 x 3.1: 15 0,0
SOT95P280X145-5N = smd 1.2 x 0.6: 1 -1.25,0.95; 2 -1.25,0; 3 -1.25,-0.95; 4 1.25,-0.95; 5 1.25,0.95
SON50P300X300X90-13N = smd 0.8 x 0.25: 1 -1.5,1.25; 2 -1.5,0.75; 3 -1.5,0.25; 4 -1.5,-0.25; 5 -1.5,-0.75; 6 -1.5,-1.25; 7 1.5,-1.25; 8 1.5,-0.75; 9 1.5,-0.25; 10 1.5,0.25; 11 1.5,0.75; 12 1.5,1.25 | smd 1.75 x 2.45: 13 0,0
HDRV2W66P0X254_1X2_508X249X106 = drill 1.15 pad 1.725 square: 1 0,0 | drill 1.15 pad 1.725: 2 2.54,0
878980666 = smd 1.27 x 2.96: 1 -6.35,1.79; 2 -3.81,-1.79; 3 -1.27,1.79; 4 1.27,-1.79; 5 3.81,1.79; 6 6.35,-1.79
39532104 = drill 0.85 pad 1.381 square: 1 0,0 | drill 0.85 pad 1.381: 2 1.25,5; 3 2.5,0; 4 3.75,5; 5 5,0; 6 6.25,5; 7 7.5,0; 8 8.75,5; 9 10,0; 10 11.25,5
INDC3030X155N = smd 1.4 x 3.2: 1 -1.25,0; 2 1.25,0
XAL40XX = smd 0.98 x 3.4: 1 -1.185,0; 2 1.185,0
LEDC1006X25N = smd 0.7 x 0.7: 1 -0.55,0; 2 0.55,0
FMMT619TA = smd 0.8 x 0.9: 1 -0.95,-0.85; 2 0.95,-0.85; 3 0,1.15
RESC1005X40N = smd 0.75 x 0.6: 1 -0.55,0; 2 0.55,0
RESC1608X55N = smd 0.9 x 1: 1 -0.8,0; 2 0.8,0
JS202011SCQN = smd 1.2 x 2.5: 1 -2.5,-2.75; 2 0,-2.75; 3 2.5,-2.75; 4 -2.5,2.75; 5 0,2.75; 6 2.5,2.75
SKRPADE010 = smd 1.05 x 0.65: 1 -1.95,1.075; 2 2.2,1.075; 3 -1.95,-1.075; 4 2.2,-1.075
SMTU2032LF = smd 2.6 x 3.5: 1 -14.7,0; 2 14.7,0
3224W1205E = smd 1.6 x 1.3: 1 1.45,-1.27; 3 1.45,1.23 | smd 1.6 x 2: 2 -1.45,-0.02

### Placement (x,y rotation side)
C1  6.86,12.83 90 top
C2  2.92,13.08 90 top
C3  2.41,19.43 90 top
C4  7.87,19.43 90 top
C5  7.87,23.24 90 top
C6  24.13,55.12 0 top
C7  24.13,56.39 0 top
C8  18.67,47.5 90 top
C9  20.95,45.34 180 top
C10  8.76,57.53 270 top
C11  8.13,55.63 180 bottom
C12  6.6,57.66 90 bottom
C13  3.3,55.24 0 bottom
C14  4.95,54.74 90 bottom
C15  6.86,60.58 90 bottom
C16  22.23,47.12 90 top
C17  23.37,47.12 90 top
C18  16.64,42.67 0 bottom
C19  14.48,31.88 180 bottom
C20  14.48,33.53 180 bottom
C21  21.08,40.89 90 bottom
C22  23.5,42.04 270 bottom
C23  13.97,41.78 90 bottom
D1  22.23,36.32 270 bottom
IC1  5.33,19.43 90 top
IC2  23.75,51.69 0 top
IC3  7.49,53.98 90 top
IC4  9.78,58.93 90 bottom
IC5  3.81,58.04 90 bottom
IC6  16.76,39.75 270 bottom
J1  5.08,27.18 180 top
J2  17.27,55.75 180 top
J3  17.27,59.18 180 top
J4  14.73,52.32 0 top
J5  18.41,39.88 180 top
J6  19.56,68.71 180 top
J7  5.08,30.61 180 top
L1  4.06,23.24 0 top
L2  17.78,34.8 0 bottom
LED1  26.54,47.88 0 top
LED2  9.91,59.69 0 top
LOGO_CMUA  [CMUA_4.5X5.5]  17.65,6.86 0 bottom
LOGO_ICN2  [ICN2_5.59X3.47]  11.68,6.35 0 bottom
Q1  12.7,48.13 0 bottom
Q2  10.92,43.81 0 bottom
R1  5.84,16.89 0 top
R2  5.84,15.62 180 top
R3  20.07,50.04 90 top
R4  20.07,47.5 270 top
R5  27.3,50.8 270 top
R6  9.91,57.53 90 top
R7  11.18,57.53 90 top
R8  12.32,54.86 90 bottom
R9  9.27,53.85 270 bottom
R10  11.05,53.85 270 bottom
R11  4.95,60.96 0 bottom
R12  14.22,45.34 180 bottom
R13  9.4,47.24 180 bottom
R14  13.97,35.81 90 bottom
R15  19.56,39.5 270 bottom
R16  18.67,31.75 180 bottom
R17  17.02,29.97 0 bottom
R18  19.56,42.67 270 bottom
R19  13.97,39.12 90 bottom
S1  4.83,5.97 90 top
S2  14.35,47.5 0 top
U1  18.8,18.16 90 top
VR1  3.94,43.69 0 top

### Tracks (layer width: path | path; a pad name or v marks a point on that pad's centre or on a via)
3.0V
  Top 0.152: C4.2 7.87,21.08 6.99,21.97 6.99,23.41 7.37,23.79 C5.2 7.87,24.89 5.59,27.18 J1.1 | IC1.4 7.62,20.38 C4.2 | C4.2 7.87,20.03 6.92,19.07 6.92,17.42 R1.2
28.6V  (via drill 0.3)
  Top 0.152: v27.01,40.51 v24.89,40.51
  Bottom 0.152: R15.2 21.9,38.7 | 21.9,38.7 22.17,38.43 | 22.17,38.43 D1.1 24,36.59 24,32.77 23.11,31.88 19.6,31.88 R16.2 | 22.17,38.43 23.5,39.75 C22.2 23.57,40.51 v24.89,40.51 | C21.1 21.08,39.52 21.9,38.7 | J6.2 18.31,67.46 J6.1 24.64,68.71 28.23,65.12 28.23,41.56 27.18,40.51 v27.01,40.51
A
  Bottom 0.152: Q1.1 13.67,47.26 R12.1 12.57,45.34 12.2,44.97 Q2.3
B
  Bottom 0.152: Q1.2 9.99,47.28 R13.2 9.95,44.41 10.29,44.07 11.3,44.07 11.87,43.5 Q2.1
BAT
  Top 0.152: U1.1 18.8,6.35 16.68,8.47 S1.3 S1.6
C  (via drill 0.35)
  Top 0.152: VR1.2 4.14,43.67 VR1.1 7.75,42.42 v8.38,43.05
  Bottom 0.152: R13.1 8.38,46.78 v8.38,43.05
CATHODE  (via drill 0.3, 0.35)
  Top 0.152: v8.89,49.28 8.38,48.77 v6.86,48.77
  Bottom 0.152: J6.9 8.31,67.46 J6.10 7.39,62.79 3.71,62.79 1.93,61.01 1.93,53.7 v6.86,48.77 | Q1.3 v8.9,49.28 v8.89,49.28
CE  (via drill 0.35)
  Top 0.152: v12.57,61.47 12.57,61.94 J6.8
  Bottom 0.152: J6.7 10.81,67.46 J6.8 | IC4.14 11.98,60.88 v12.57,61.47
COMP
  Bottom 0.152: R19.1 14.04,38.25 IC6.12
COMP*
  Bottom 0.152: R19.2 C23.1
FB1
  Top 0.152: IC1.2 5.33,16.97 | 5.33,16.97 5.33,15.66 R2.2 | 5.33,16.97 R1.1
FB2
  Bottom 0.152: IC6.3 16.51,41.78 16.73,42.01 18.23,42.01 18.37,41.87 R18.2 | R18.2 R15.1 | R18.2 20.65,41.87 C21.2
GND  (via drill 0.35)
  Top 0.152: C2.1 2.93,11.68 6.26,11.68 C1.1 7.87,13.29 v7.87,16.64 | IC1.3 5.98,19.16 5.71,19.43 3.11,19.43 C3.1 2.41,17.4 v2.54,17.27 | 18.8,32.64 U1.2 19.68,33.75 J5.3 | 18.8,32.64 18.8,26.92 13.72,21.84 8.76,21.84 | v23.37,45.21 21.71,45.21 C9.1 20.48,44.42 19.85,44.42 19.56,44.7 19.56,46.06 C8.1 17.99,46.95 17.47,46.42 S2.4 S2.3 6.89,46.42 VR1.3 1.99,48.31 IC3.2 | v23.37,45.21 25.99,47.84 LED1.1 26.07,47.88 26.65,47.3 27.54,47.3 | IC3.13 4.39,59 4.7,59.31 6.22,59.31 6.35,59.18 v6.86,59.18 7.66,59.18 C10.1 | 8.76,21.84 8.76,19.62 C4.1 v7.87,16.64 | 8.76,21.84 7.92,22.69 C5.1 | R2.1 7.41,16.64 v7.87,16.64 | v13.21,57.4 24.13,57.4 24.58,56.95 C7.2 24.68,56.29 C6.2 24.72,55.07 IC2.13 27.13,53.64 27.94,52.83 27.94,47.7 27.54,47.3 | 27.54,47.3 27.54,35.41 24.77,32.64 18.8,32.64 | C16.1 C17.1 v23.37,45.21
  Bottom 0.152: 13.41,39.12 14.61,39.12 15.24,39.75 IC6.13 17.01,40 IC6.4 IC6.5 IC6.6 | 13.41,39.12 13.34,39.12 12.32,38.1 12.32,36.07 13.34,35.05 13.93,35.05 R14.1 13.93,34.97 C20.1 13.78,33.38 C19.1 13.78,31.05 14.86,29.97 R17.2 | 12.83,56.39 12.24,56.98 IC4.1 11.28,57.43 IC4.15 8.28,57.43 IC4.7 7.83,56.98 7.58,56.73 | 12.83,56.39 12.85,56.37 12.85,54.84 R8.1 | 7.58,56.73 C11.1 6.24,54.29 C14.1 4.81,54.29 C13.1 3.85,56.75 IC5.2 3.81,57.66 4.19,58.04 4.95,58.04 5.46,58.55 5.46,59.69 5.8,60.03 C15.1 v6.86,59.18 | C12.1 7.1,57.21 7.58,56.73 | v2.54,17.27 7.24,17.27 v7.87,16.64 | v23.37,45.21 23.5,45.09 C22.1 23.33,43.47 R18.1 18.58,43.47 17.91,42.8 17.31,42.8 C18.1 17.19,43.14 16.89,43.43 14.1,43.43 13.97,43.31 C23.2 13.8,42.16 13.11,42.16 | Q2.2 10.77,42.16 13.11,42.16 | v13.21,57.4 12.83,57.02 12.83,56.39 | 13.11,42.16 13.11,39.47 13.41,39.17 13.41,39.12
  pour Top (isolate 0.254): 0,70.1 28.7,70.1 28.7,0 0,0 0,48.77 6.22,48.77 6.22,50.29 8.26,50.29 8.26,57.66 6.1,57.66 6.1,59.18 0,59.18
  pour Bottom (isolate 0.254): 0,70.1 28.7,70.1 28.7,0 0,0
IC3_RX  (via drill 0.3)
  Top 0.152: IC3.7 8.15,52.17 8.5,51.82 v8.5,51.81
  Bottom 0.152: v8.5,51.81 8.53,51.78 11.47,51.78 14.73,55.04 J2.2
IC3_TX  (via drill 0.3)
  Top 0.152: v8.51,52.57 7.7,53.38 IC3.8
  Bottom 0.152: v8.51,52.57 8.64,52.44 11.44,52.44 13.15,54.15 13.15,56.2 14.73,57.78 J3.2
IC5_OUT
  Bottom 0.152: R11.2 4.4,59.65 IC5.5
IC5_REF
  Bottom 0.152: IC5.1 4.95,56.6 C14.2
IC6_VIN  (via drill 0.35)
  Top 0.152: J7.1 5.21,30.73 15.75,30.73 v16.26,31.24
  Bottom 0.152: IC6.10 16.51,34.88 L2.2 15.32,33.53 C20.2 15.18,33.38 C19.2 15.81,31.88 16.26,31.43 v16.26,31.24
ICSPCLK  (via drill 0.3)
  Top 0.152: IC2.11 26.49,52.01 v26.8,52.32 | v26.16,44.7 25.53,44.07 16,44.07 14.61,42.67 J5.5
  Bottom 0.152: v26.8,52.32 27.18,52.32 27.43,52.07 27.43,45.97 v26.16,44.7
ICSPDAT  (via drill 0.3)
  Top 0.152: IC2.12 26.12,53.09 v26.93,53.09 v26.94,53.08 | v26.16,43.69 19.16,43.69 J5.4
  Bottom 0.152: v26.94,53.08 27.92,52.1 27.92,45.45 v26.16,43.69
ION  (via drill 0.35)
  Top 0.152: v12.98,37.59 12.98,42.57 v14.73,44.32
  Bottom 0.152: IC6.11 16.01,37.6 15.02,36.61 R14.2 13.42,36.61 12.98,37.06 v12.98,37.59 | J4.1 14.73,45.38 | 14.73,45.38 R12.2 | v14.73,44.32 14.73,45.38
L
  Top 0.152: L1.2 5.31,20.4 IC1.5
LED1
  Top 0.152: LED1.2 27.3,48.09 R5.2
LED2_K
  Top 0.152: LED2.1 9.91,59.14 R6.2
LED_STATE
  Top 0.152: IC2.10 25.71,51.35 R5.1
MEMB
  Bottom 0.152: IC4.2 10.78,56.4 11.05,56.13 12.06,56.13 12.32,55.88 R8.2
N$1
  Top 0.152: 0,70.1 28.7,70.1 28.7,0 0,0 0,70.1
N$2
  Bottom 0.152: 0,70.1 28.7,70.1 28.7,0 0,0 0,70.1
OVP
  Bottom 0.152: IC6.9 17.01,37.47 17.87,36.61 R16.1 17.82,31.7 R17.1
P0_2
  Top 0.152: IC3.12 5.65,58.17 7.62,58.17 8.24,57.55 9.29,57.55 9.86,56.98 R6.1
P2_0  (via drill 0.35)
  Top 0.152: J5.6 11.04,40.64 1.91,40.64 1.14,41.4 v1.14,43.94 | v0.73,60.07 0.48,59.82 0.48,58.54 IC3.16
  Bottom 0.152: v1.14,43.94 1.14,59.82 0.89,60.07 v0.73,60.07
RC4
  Top 0.152: J4.2 17.91,51.69 20.06,51.69 20.64,51.11 20.64,50.57 21.48,49.73 22.76,49.73 IC2.5
RE
  Bottom 0.152: IC4.13 10.79,60.89 10.79,61.59 11.3,62.1 14.2,62.1 15.74,63.64 | 15.74,63.64 J6.4 | J6.3 15.74,67.39 15.74,63.64
RST_N
  Top 0.152: C10.2 7.56,55.77 IC3.10 9.95,55.77 11.16,56.98 R7.1
RX  (via drill 0.3)
  Top 0.152: v20.7,52.83 v20.71,52.83 21.53,52.01 IC2.2
  Bottom 0.152: J3.1 17.27,58.04 15.88,56.64 15.88,54.86 16.51,54.23 19.3,54.23 v20.7,52.83
S2
  Top 0.152: R3.1 R4.1 C8.2 17.99,48.05 17.47,48.57 S2.2 16.38,48.57 S2.1
SCL  (via drill 0.3)
  Top 0.152: v25.6,49.99 25.6,50.6 IC2.9 | v22.25,54.71 18.29,54.71 18.14,54.56 12.04,54.56 v11.28,55.32
  Bottom 0.152: IC4.3 10.28,55.68 10.96,55 | R10.1 11.05,54.91 10.96,55 | v25.6,49.99 25.6,51.36 v22.25,54.71 | 10.96,55 v11.28,55.32
SDA  (via drill 0.3)
  Top 0.152: v20.88,47.09 23.77,47.09 24.69,48.01 24.69,49.68 IC2.8 | v17.07,50.9 13.11,50.9 v10.06,53.95
  Bottom 0.152: IC4.4 9.78,56.34 9.27,55.84 R9.1 9.72,53.95 v10.06,53.95 | v17.07,50.9 v20.88,47.09
SS
  Bottom 0.152: IC6.2 16.01,42.6 C18.2
SW
  Bottom 0.152: D1.2 19.49,34.27 L2.1 18.96,36.79 18.01,37.74 IC6.7 IC6.8
TX  (via drill 0.3)
  Top 0.152: IC2.1 20.74,53.72 v20.7,53.72
  Bottom 0.152: J2.1 18.49,54.53 19.81,54.53 20.62,53.72 v20.7,53.72
VDD  (via drill 0.3, 0.35)
  Top 0.152: IC2.16 22.77,54.31 C6.1 23.68,55.22 C7.1 21.59,56.39 v21.21,56.77 | J1.2 J7.2 7.11,35.18 v7.24,35.18 16,35.18 17.4,36.58 17.4,38.35 20.71,41.67 J5.2 24.27,41.67 24.89,42.29 v24.89,42.8 | v2.92,60.83 3.19,60.56 | 3.19,60.56 IC3.14 | 3.19,60.56 9.59,60.56 LED2.2 10.46,58.8 R7.2 21.06,58.08 v21.21,57.94 | R4.2 20.07,46.35 | 20.07,46.35 20.07,45.53 C9.2 | v21.08,46.35 20.07,46.35
  Bottom 0.152: IC4.6 8.78,55.73 C11.2 8.72,55.58 8.72,53.72 | 7.75,53.72 7.75,38.61 7.24,38.1 v7.24,35.18 | v2.92,60.83 2.92,59.35 IC5.4 IC5.3 2.86,55.35 C13.2 4.28,53.72 7.75,53.72 | v24.89,42.8 24.89,44.7 23.75,45.85 21.59,45.85 v21.08,46.35 | 7.75,53.72 8.72,53.72 | v21.21,57.94 v21.21,56.77 | R10.2 R9.2 9.14,53.3 8.72,53.72
VIN
  Top 0.152: S1.2 S1.5 0.68,5.97 0.51,6.14 0.51,13.34 1.66,14.49 C2.2 | C2.2 5.74,14.49 C1.2 | L1.1 2.81,21.36 | 2.81,21.36 2.41,20.95 C3.2 1.84,20.13 1.27,19.56 1.27,17.44 2.92,15.79 | 2.81,21.36 3.79,20.38 IC1.6 | 2.92,15.79 C2.2 | 2.92,15.79 2.94,15.77 4.06,16.89 4.06,17.86 IC1.1
VOUT  (via drill 0.3)
  Top 0.152: v8.76,61.85 11.05,61.85 12.57,60.33 19.18,60.33 20.07,59.44 v20.07,58.93 | v23.9,48.51 24.07,48.69 IC2.7
  Bottom 0.152: C12.2 6.93,58.11 7.49,58.67 7.49,60.09 IC4.8 8.28,61.62 8.51,61.85 v8.76,61.85 | v20.07,58.93 20.07,56.13 21.84,54.36 21.84,48.9 22.23,48.51 v23.9,48.51
VPP/*MCLR  (via drill 0.3)
  Top 0.152: J5.1 26.04,39.36 v26.04,39.37 | IC2.3 21.35,51.36 v20.7,52.02 | R3.2 20.02,50.55 v19.18,50.55
  Bottom 0.152: v26.04,39.37 26.04,42.8 25.2,43.64 25.2,44.83 23.88,46.15 22.68,46.15 19.18,49.66 v19.18,50.55 19.18,51.44 19.76,52.02 v20.7,52.02
VREF  (via drill 0.3)
  Top 0.152: IC2.6 23.37,49.68 C17.2 C16.2 22.1,47.7 v21.34,48.46 | v11.89,60.2 10.97,60.2 9.91,61.27 8.53,61.27 8.23,61.57 v8.23,62.48
  Bottom 0.152: R11.1 6.69,60.96 C15.2 6.86,61.89 7.45,62.48 v8.23,62.48 9.21,62.48 9.78,61.91 IC4.11 | v21.34,48.46 21.34,54.41 18.44,57.3 18.44,60.2 18.29,60.35 12.04,60.35 v11.89,60.2
WE
  Bottom 0.152: IC4.12 10.4,61 10.4,61.63 11.18,62.41 12.19,62.41 13.31,63.52 J6.6 13.31,67.46 J6.5

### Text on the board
tPlace: 1 | RX | BLE | TX | ION | STATE | bS2 | v1.0 | System | BOOST | BAT | ON
bPlace: K | CE | WE | RE | A | v1.0 | bS2·System | Miguel A. Aroca | Giulio Rosati | Johann F. Osma | Arben Merkoçi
